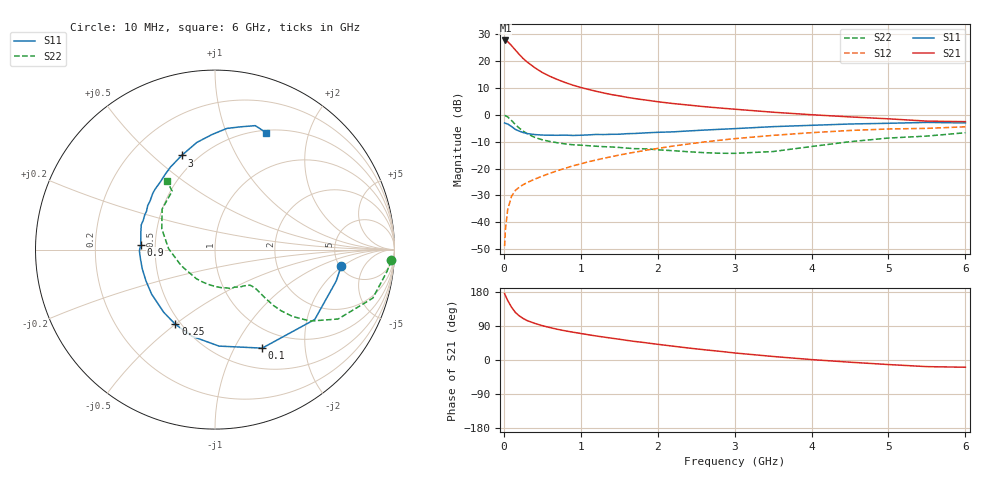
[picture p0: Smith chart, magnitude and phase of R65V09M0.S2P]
! SIEMENS Small Signal Semiconductors
! BFR193
! Si NPN RF Bipolar Junction Transistor in SOT23
! VCE = 5 V  IC = 9 mA
! Common Emitter S-Parameters:  May  1996
# GHz  S  MA  R  50
!  f  S11  S21  S12  S22
! GHz  MAG  ANG  MAG  ANG  MAG  ANG  MAG  ANG
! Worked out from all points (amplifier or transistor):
!   36 points, 10 MHz to 6 GHz, reference 50 ohm
!   highest |S21| = 27.7 dB at 20 MHz (marker M1)
!   |S21| within 3 dB of that: start of sweep to 132.6 MHz
!   unconditionally stable (mu >= 1): 775.8 MHz to 2.008 GHz
!   at 250 MHz: K = 0.60, MSG = 23.5 dB, |S12| = -26.0 dB
!   at 1.4 GHz: K = 1.04, MAG = 10.3 dB, |S12| = -15.5 dB
!   at 6 GHz: K = 0.95, MSG = 1.0 dB, |S12| = -4.4 dB
!   S11 on the Smith chart (normalised r, x): 10 MHz: 5.16, -1.90; 100 MHz: 0.75, -1.30; 250 MHz: 0.47, -0.50; 900 MHz: 0.41, +0.03; 3 GHz: 0.41, +0.62; 6 GHz: 0.53, +1.40
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0.01  0.7092 -7.4  24.28 175.3  0.0036 87.3  0.9836 -3.5
0.02  0.6978 -14.5  24.4 170.2  0.0072 84.8  0.9669 -7.1
0.05  0.6786 -35.0  23.15 157.1  0.0173 74.2  0.9198 -17.1
0.1  0.6087 -64.4  19.55 139.3  0.0305 64.6  0.7876 -29.4
0.15  0.5381 -87.6  16.17 125.6  0.0394 57.9  0.6633 -36.9
0.2  0.4998 -104.8  13.42 116.5  0.045 55.6  0.5693 -40.8
0.25  0.4713 -117.9  11.3 109.7  0.0502 54.3  0.5013 -42.8
0.3  0.4514 -129.2  9.769 104.3  0.0547 54.7  0.45 -43.7
0.4  0.4316 -145.0  7.629 96.8  0.0637 56.1  0.3833 -44.0
0.5  0.4221 -155.8  6.171 90.6  0.0725 58.1  0.3445 -43.8
0.6  0.4192 -165.0  5.234 85.5  0.0822 59.2  0.3204 -43.7
0.7  0.4184 -172.4  4.547 80.9  0.092 60.5  0.3027 -44.2
0.9  0.4148 176.2  3.58 73.3  0.1129 61.9  0.2784 -45.5
1.1  0.4254 166.1  2.986 66.6  0.1342 62.1  0.2675 -48.7
1.3  0.4318 157.7  2.564 60.5  0.1564 61.8  0.2568 -52.3
1.6  0.4481 146.8  2.132 51.8  0.1907 60.2  0.2414 -59.8
2.2  0.4845 129.0  1.631 36.5  0.2635 55.0  0.2159 -79.8
3  0.5564 109.5  1.28 18.6  0.3618 44.7  0.1927 -122.1
3.5  0.6057 99.6  1.124 9.3  0.4167 37.2  0.2083 -154.4
4.5  0.6785 84.4  0.92 -5.8  0.5141 22.2  0.3179 158.8
5.5  0.7262 72.0  0.768 -17.5  0.5625 6.5  0.404 126.2
6  0.7108 66.2  0.75 -19.1  0.6011 1.9  0.4663 125.0
